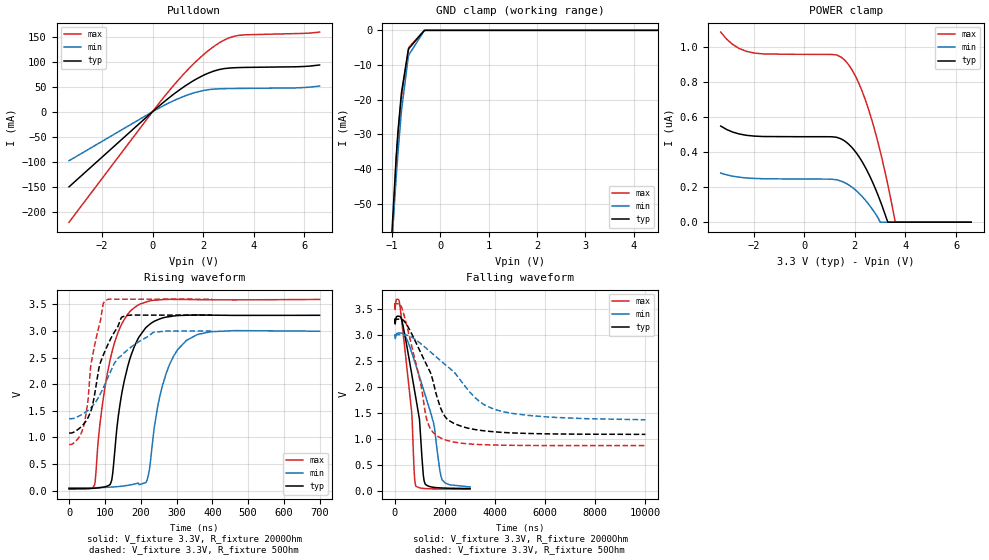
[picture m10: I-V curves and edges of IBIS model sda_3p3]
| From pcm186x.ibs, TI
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|   sda_3p3 Model
[Model]   sda_3p3
Model_type   I/O_open_drain
Polarity   Non-Inverting
Vinl = 0.99
Vinh = 2.31
Vmeas = 1.65
Vref = 3.3
Cref = 400pF
Rref = 2000
|   typ   min   max
|   (nom PVT)   (fast PVT)   (slow PVT)
C_comp   9.782e-12   9.782e-12   9.904e-12
[Model spec]
|subparameter
Vinl   0.99   0.9   1.08
Vinh   2.31   2.1   2.52
| Where nom  PVT is Nominal Process, 3.3V, 27C
|   Fast PVT is Strong Process,  3.6V, -40C
|   Slow PVT is Weak Process,   3V, 125C
[Voltage Range]   3.3   3   3.6
|Junction Temperature
[Temperature Range]   27   125   -40
[Pullup Reference]   3.3   3   3.6
[Pulldown Reference]   0   0   0
[Power Clamp Reference]   3.3   3   3.6
[GND Clamp Reference]   0   0   0
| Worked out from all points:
|   slope of the pulldown table from 0 to 0.495 V, typ, clamps not added: 23.1 ohm
|   falling waveform, V_fixture 3.3V, R_fixture 2000Ohm: 20-80 % time 546ns typ, 881ns min, 375ns max; typ from 3.3 V to 0.04 V
|   rising waveform, V_fixture 3.3V, R_fixture 2000Ohm: 20-80 % time 51.7ns typ, 54.4ns min, 52.7ns max; typ from 0.036 V to 3.3 V
|   falling waveform, V_fixture 3.3V, R_fixture 50Ohm: 20-80 % time 1.05us typ, 2.04us min, 713ns max; typ from 3.3 V to 1.08 V
|   rising waveform, V_fixture 3.3V, R_fixture 50Ohm: 20-80 % time 53.8ns typ, 92.1ns min, 35.5ns max; typ from 1.08 V to 3.3 V
[Pulldown]
|   Voltage   I(typ)   I(min)   I(max)
-3.3V     -150.4mA   -98.16mA   -221.2mA
459mV     19.98mA    12.77mA    29.8mA
917.4mV   38.25mA    24mA       57.66mA
1.464V    57.39mA    34.94mA    87.9mA
1.971V    71.88mA    42.05mA    112.4mA
2.391V    80.81mA    45.12mA    129.5mA
2.862V    86.48mA    46.15mA    144.2mA
3.4V      88.34mA    46.55mA    152.7mA
5.637V    89.93mA    47.63mA    156.4mA
6.6V      93.49mA    51.3mA     159.4mA
[GND Clamp]
|   Voltage   I(typ)   I(min)   I(max)
-3.3V     -1.428A    -1.177A    -1.713A
-1.05V    -70.15mA   -71.58mA   -76.36mA
-916.8mV  -37.28mA   -42.97mA   -38.23mA
-897mV    -33.16mA   -39.12mA   -33.94mA
-874.5mV  -28.81mA   -34.91mA   -29.62mA
-805.2mV  -18.02mA   -23.25mA   -19.29mA
-666.6mV  -6.002mA   -7.943mA   -5.783mA
-654mV    -5.286mA   -7.093mA   -4.946mA
-330mV    -4.474uA   -40.92uA   -707.9nA
6.6V      0A         0A         0A
[POWER Clamp]
|   Voltage   I(typ)   I(min)   I(max)
-3.3V     548.4nA    280.3nA    1.085uA
-2.828V   514.4nA    262.6nA    1.014uA
-1.986V   491.3nA    249.7nA    965.5nA
1.096V    487.3nA    245.1nA    957nA
1.53V     469.6nA    230.1nA    933.6nA
2.046V    397.8nA    181.1nA    827.2nA
2.303V    341.4nA    144.3nA    741.6nA
2.571V    268.7nA    97.75nA    630.3nA
3.003V    121.8nA    0A         404.4nA
3.303V    0A         0A         214.2nA
3.598V    0A         0A         0A
6.6V      0A         0A         0A
[Ramp]
R_load = 2000
|   typ   min   max
dV/dt_r   1.95616/5.13949e-08   1.76827/5.41553e-08   2.14077/5.26293e-08
dV/dt_f   1.95551/5.4566e-07   1.75694/8.80094e-07   2.14231/3.74345e-07
[Falling Waveform]
V_fixture = 3.3V
V_fixture_min = 3V
V_fixture_max = 3.6V
R_fixture = 2000Ohm
|   Time   V(typ)   V(min)   V(max)
0s        3.299V     3V         3.598V
154.6ns   3.358V     3.034V     3.677V
268.7ns   3.294V     3.032V     3.289V
679.7ns   2.222V     2.648V     1.452V
773.4ns   1.96V      2.51V      336.4mV
835.2ns   1.787V     2.418V     83.67mV
1.21us    125.3mV    1.839V     38.95mV
1.546us   63.17mV    1.299V     32.56mV
1.89us    50.1mV     203.7mV    30.03mV
3us       39.84mV    71.27mV    27.56mV
[Rising Waveform]
V_fixture = 3.3V
V_fixture_min = 3V
V_fixture_max = 3.6V
R_fixture = 2000Ohm
|   Time   V(typ)   V(min)   V(max)
0s        36.23mV    50.58mV    26.78mV
71.6ns    44.66mV    53.83mV    111.7mV
86.2ns    54.7mV     56.82mV    1.251V
114.5ns   112.5mV    65.06mV    2.454V
146.2ns   1.788V     81.25mV    3.121V
182.5ns   2.712V     123.4mV    3.439V
216ns     3.074V     163.6mV    3.549V
260.8ns   3.246V     1.976V     3.592V
327.7ns   3.297V     2.824V     3.594V
699.3ns   3.296V     2.998V     3.595V
[Falling Waveform]
V_fixture = 3.3V
V_fixture_min = 3V
V_fixture_max = 3.6V
R_fixture = 50Ohm
|   Time   V(typ)   V(min)   V(max)
0s        3.3V       3V         3.6V
207ns     3.301V     3.001V     3.591V
352ns     3.274V     3V         3.403V
1.04us    2.648V     2.827V     2.039V
1.306us   2.382V     2.718V     1.313V
1.754us   1.693V     2.531V     1.032V
2.362us   1.292V     2.283V     934.5mV
3.186us   1.177V     1.797V     891.8mV
3.94us    1.133V     1.57V      877.7mV
9.999us   1.083V     1.364V     866.6mV
[Rising Waveform]
V_fixture = 3.3V
V_fixture_min = 3V
V_fixture_max = 3.6V
R_fixture = 50Ohm
|   Time   V(typ)   V(min)   V(max)
0s        1.082V     1.352V     866.5mV
25ns      1.15V      1.393V     976.6mV
42ns      1.259V     1.457V     1.247V
53ns      1.373V     1.51V      1.708V
61ns      1.498V     1.558V     2.364V
85ns      2.354V     1.79V      3.128V
99ns      2.604V     1.982V     3.556V
148ns     3.265V     2.552V     3.6V
235ns     3.3V       2.976V     3.6V
399ns     3.3V       3V         3.6V
